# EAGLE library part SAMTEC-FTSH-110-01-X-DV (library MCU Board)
Buy Part
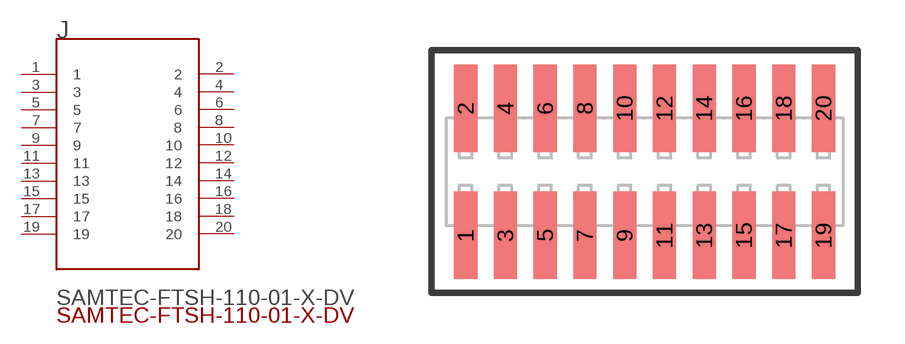
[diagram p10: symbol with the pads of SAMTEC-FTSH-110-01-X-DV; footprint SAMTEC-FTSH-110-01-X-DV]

Designator prefix J

## SAMTEC-FTSH-110-01-X-DVJ (AVAILABILITY: Bad; DESCRIPTION: FTSH Series .050 Micro Terminal Strip; MF: Samtec; MP: FTSH-110-01-S-DV; PACKAGE: None; PRICE: None)  [SAMTEC-FTSH-110-01-X-DV]
1  1  pas
2  2  pas
3  3  pas
4  4  pas
5  5  pas
6  6  pas
7  7  pas
8  8  pas
9  9  pas
10  10  pas
11  11  pas
12  12  pas
13  13  pas
14  14  pas
15  15  pas
16  16  pas
17  17  pas
18  18  pas
19  19  pas
20  20  pas

## Footprint SAMTEC-FTSH-110-01-X-DV (pad centres in mm)
translated Allegro footprint
smd 0.74 x 2.79: 1 -5.715,-2.032; 2 -5.715,2.032; 3 -4.445,-2.032; 4 -4.445,2.032; 5 -3.175,-2.032; 6 -3.175,2.032; 7 -1.905,-2.032; 8 -1.905,2.032; 9 -0.635,-2.032; 10 -0.635,2.032; 11 0.635,-2.032; 12 0.635,2.032; 13 1.905,-2.032; 14 1.905,2.032; 15 3.175,-2.032; 16 3.175,2.032; 17 4.445,-2.032; 18 4.445,2.032; 19 5.715,-2.032; 20 5.715,2.032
